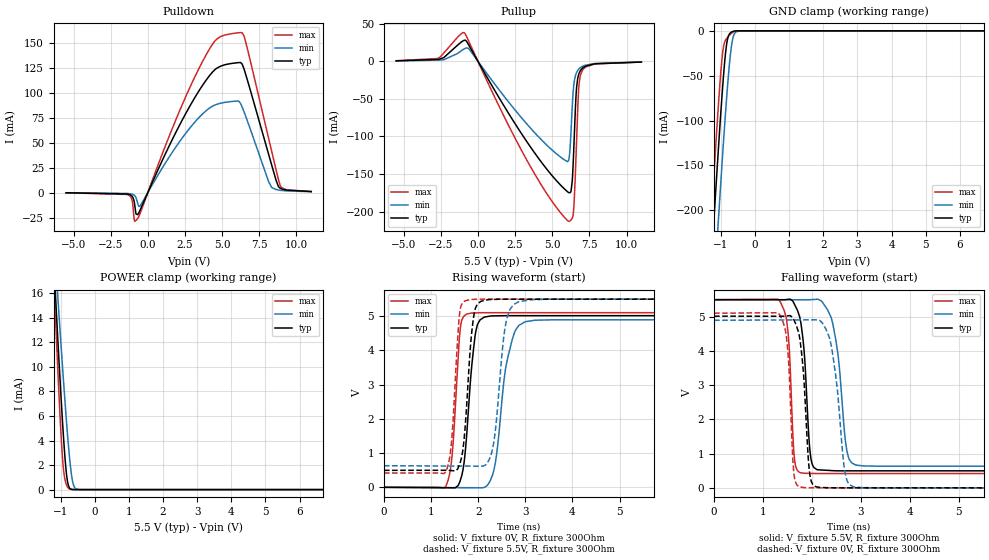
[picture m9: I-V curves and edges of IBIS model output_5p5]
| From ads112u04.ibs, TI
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|   output_5p5 Model
[Model]   output_5p5
Model_type   3-state
Polarity   Non-Inverting
Vmeas = 2.75
Vref = 0
Cref = 2pF
Rref = 100000
|   typ   min   max
C_comp   1.30508E-12   1.28718E-12   1.31102E-12
|C_comp_pullup   1.00589E-12   9.63036E-13   1.01301E-12
|C_comp_pulldown   9.94586E-13   9.76393E-13   9.94602E-13
| Where Nom  PVT is Nominal Process, 5.5V, 27C
|   Fast PVT is Strong Process,  5.501V, -40C
|   Slow PVT is Weak Process,   5.499, 125C
[Voltage Range]   5.5   5.499   5.501
[Temperature Range]   27   125   -40
[Pullup Reference]   5.5   5.499   5.501
[Pulldown Reference]   0   0   0
[Power Clamp Reference]   5.5   5.499   5.501
[GND Clamp Reference]   0   0   0
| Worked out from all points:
|   slope of the pulldown table from 0 to 0.825 V, typ, clamps not added: 30.1 ohm
|   slope of the pullup table from 0 to 0.825 V, typ, clamps not added: 29 ohm
|   GND clamp passes 1 mA (typ) near -0.67 V on its own axis
|   POWER clamp passes 1 mA (typ) near -0.82 V on its own axis
|   falling waveform, V_fixture 5.5V, R_fixture 300Ohm: 20-80 % time 133ps typ, 205ps min, 99.1ps max; typ from 5.5 V to 0.497 V
|   rising waveform, V_fixture 0V, R_fixture 300Ohm: 20-80 % time 176ps typ, 258ps min, 136ps max; typ from 0 V to 5.02 V
|   rising waveform, V_fixture 5.5V, R_fixture 300Ohm: 20-80 % time 154ps typ, 196ps min, 131ps max; typ from 0.497 V to 5.5 V
|   falling waveform, V_fixture 0V, R_fixture 300Ohm: 20-80 % time 136ps typ, 208ps min, 101ps max; typ from 5.02 V to 0 V
[Pulldown]
|   Voltage   I(typ)   I(min)   I(max)
-5.5V     -139.3uA   -99uA      -151.9uA
-1.375V   -1.389mA   -809.8uA   -1.837mA
-995.5mV  -5.057mA   -1.916mA   -13.95mA
-797.5mV  -21.26mA   -4.804mA   -27.93mA
-517mV    -17.41mA   -13.25mA   -20.88mA
3.938V    112.8mA    82.15mA    138.3mA
4.862V    126.3mA    89.35mA    155.9mA
6.248V    130.2mA    89.06mA    160.2mA
6.495V    122.9mA    80.2mA     155.9mA
8.129V    38.5mA     11.1mA     54.46mA
8.921V    4.291mA    2.335mA    6.879mA
11V       1.086mA    904uA      1.089mA
[GND Clamp]
|   Voltage   I(typ)   I(min)   I(max)
-5.5V     -3.028A    -3.1A      -2.983A
-1.359V   -306.6mA   -386.8mA   -256.2mA
-1.243V   -234.4mA   -314.6mA   -184mA
-1.21V    -214.1mA   -294.2mA   -163.7mA
-1.078V   -134.5mA   -213.7mA   -85.66mA
-946mV    -61.19mA   -136.2mA   -23.55mA
-880mV    -30.84mA   -99.67mA   -11.65mA
-814mV    -10.82mA   -65.68mA   -7.681mA
-731.5mV  -2.601mA   -29.94mA   -4.139mA
-649mV    -701.7uA   -8.211mA   -1.536mA
-385mV    -950.1nA   -10.06uA   -919.6nA
11V       0A         0A         0A
[Pullup]
|   Voltage   I(typ)   I(min)   I(max)
-5.5V     607.8uA    492.8uA    650.7uA
-2.712V   2.442mA    1.477mA    3.672mA
-913mV    27.96mA    16.59mA    37.83mA
3.311V    -107.4mA   -83.78mA   -132.1mA
6.133V    -174.7mA   -129.1mA   -212.8mA
6.199V    -174.7mA   -116.5mA   -212.2mA
6.347V    -159.6mA   -60.33mA   -208.6mA
6.479V    -103.2mA   -27.6mA    -185.7mA
6.611V    -42.84mA   -16.32mA   -121.7mA
6.776V    -17.95mA   -10.57mA   -38.71mA
7.04V     -9.011mA   -6.673mA   -11.63mA
11V       -1.024mA   -975.5uA   -1.008mA
[POWER Clamp]
|   Voltage   I(typ)   I(min)   I(max)
-5.5V     270.1mA    226mA      321.6mA
-1.21V    19.04mA    21.22mA    17.87mA
-1.144V   15.47mA    18.33mA    13.58mA
-1.078V   12mA       15.5mA     9.456mA
-995.5mV  7.867mA    12.05mA    4.792mA
-929.5mV  4.84mA     9.377mA    2.02mA
-830.5mV  1.305mA    5.597mA    391.1uA
-731.5mV  106.7uA    2.381mA    34.63uA
-682mV    25.55uA    1.2mA      7.993uA
-616mV    3.982uA    315.2uA    954.7nA
-451mV    7.318nA    3.664uA    0A
11V       0A         0A         0A
[Ramp]
R_load = 300
|   typ   min   max
dV/dt_r   3.01089/1.76048e-10   2.93831/2.58418e-10   3.06275/1.35271e-10
dV/dt_f   3.00189/1.32367e-10   2.92036/2.03848e-10   3.04962/9.88051e-11
[Falling Waveform]
V_fixture = 5.5V
V_fixture_min = 5.499V
V_fixture_max = 5.501V
R_fixture = 300Ohm
C_fixture = 0F
|   Time   V(typ)   V(min)   V(max)
0s        5.5V       5.499V     5.501V
1.356ns   5.499V     5.498V     5.424V
1.516ns   5.51V      5.498V     4.46V
1.647ns   5.351V     5.498V     790mV
1.84ns    3.983V     5.498V     426.4mV
2.014ns   658.9mV    5.504V     420.6mV
2.394ns   505.4mV    4.963V     418.9mV
2.711ns   497.6mV    1.095V     418.9mV
3.052ns   497.6mV    640.9mV    418.9mV
50ns      496.9mV    631.7mV    418.3mV
[Rising Waveform]
V_fixture = 0V
V_fixture_min = 0V
V_fixture_max = 0V
R_fixture = 300Ohm
C_fixture = 0F
|   Time   V(typ)   V(min)   V(max)
0s        -57.41nV   -71.54nV   -39.19nV
1.318ns   -12.69mV   -8.544mV   41.03mV
1.444ns   -13.91mV   -9.362mV   901.6mV
1.66ns    398.7mV    -10.77mV   4.912V
1.86ns    3.511V     -12.06mV   5.096V
1.989ns   4.772V     -12.89mV   5.101V
2.315ns   5.011V     409.6mV    5.104V
2.766ns   5.018V     4.512V     5.104V
3.212ns   5.018V     4.885V     5.104V
50ns      5.018V     4.897V     5.105V
[Rising Waveform]
V_fixture = 5.5V
V_fixture_min = 5.499V
V_fixture_max = 5.501V
R_fixture = 300Ohm
C_fixture = 0F
|   Time   V(typ)   V(min)   V(max)
0s        496.9mV    631.7mV    418.3mV
1.313ns   497.8mV    623mV      450.9mV
1.428ns   490mV      622.2mV    1.241V
1.653ns   912.8mV    620.7mV    5.355V
1.84ns    4.199V     619.5mV    5.491V
1.982ns   5.356V     618.5mV    5.497V
2.296ns   5.491V     1.072V     5.5V
2.658ns   5.499V     5.145V     5.5V
3.123ns   5.499V     5.483V     5.5V
50ns      5.5V       5.499V     5.501V
[Falling Waveform]
|Gnd
V_fixture = 0V
V_fixture_min = 0V
V_fixture_max = 0V
R_fixture = 300Ohm
C_fixture = 0F
|   Time   V(typ)   V(min)   V(max)
0s        5.018V     4.897V     5.105V
1.35ns    5.017V     4.907V     5.04V
1.504ns   5.027V     4.908V     4.03V
1.636ns   4.894V     4.909V     359.5mV
1.84ns    3.059V     4.91V      6.96mV
2.014ns   104.3mV    4.911V     2.01mV
2.357ns   3.532mV    4.38V      545.5uV
2.679ns   902.3uV    415.4mV    545.4uV
2.991ns   902uV      9.214mV    545.2uV
50ns      -57.46nV   -70.65nV   -39.33nV
